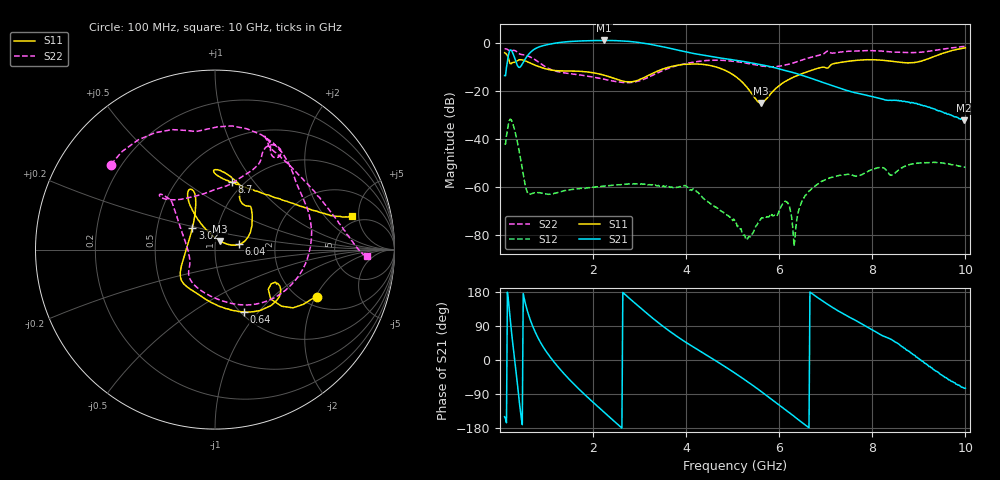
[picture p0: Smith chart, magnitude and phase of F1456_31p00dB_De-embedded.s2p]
! Integrated Device Technology
! Corporate Headquarters
! 6024 Silver Creek Valley Road
! San Jose, CA 95138  USA
! Phone:  1-408-284-8200
! Toll Free:  1-800-223-1366
! Webpage:  http://www.idt.com/
! Timing and RF Division
! 515 Groton Road, Suite 102
! Westford, MA 01886-6024
! Device:  F1456
! Description: 6-bit 0.5 dB Transmit Variable Gain Amplifier
! Frequency:  2100.0 -  2950.00 MHz
! Package:  6x6 mm Thin QFN Plastic Package: 28 pin
! State:  62
! Atten State:  31.0 dB
! Voltage:  +5.00 Volts
! Current:  216.927 mA
! Data:  The device was measured on a the F1455 evaluation board which has
!  individual transmission lines to the RF pins.  Data was collected
!  using a calibrated network analyzer.  The evaluation board was
!  de-embedded using a TRL calibration technique.
!  The reference plane is the edge of the package pin.
!  Pin  1 = CSb
!  Pin  2 = DATA
!  Pin  3 = CLK
!  Pin  4 = RSET
!  Pin  5 = GND
!  Pin  6 = RFIN  = Port 1
!  Pin  7 = GND
!  Pin  8 = NC
!  Pin  9 = NC
!  Pin 10 = NC
!  Pin 11 = NC
!  Pin 12 = NC
!  Pin 13 = NC
!  Pin 14 = /STBY
!  Pin 15 = GND
!  Pin 16 = RFOUT  = Port 2
!  Pin 17 = GND
!  Pin 18 = NC
!  Pin 19 = NC
!  Pin 20 = NC
!  Pin 21 = GND
!  Pin 22 = NC
!  Pin 23 = GND
!  Pin 24 = NC
!  Pin 25 = NC
!  Pin 26 = NC
!  Pin 27 = GND
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# GHz S dB R 50
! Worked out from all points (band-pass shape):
!   496 points, 100 MHz to 10 GHz, reference 50 ohm
!   highest |S21| = 1.01 dB at 2.24 GHz (marker M1); lowest = -32.3 dB at 9.96 GHz (marker M2)
!   |S21| within 3 dB of the highest: 802.1 MHz to 3.586 GHz (2.784 GHz wide, 127 % of centre)
!   lowest |S11| = -25.1 dB at 5.6 GHz (marker M3), VSWR 1.12, Z = 52.5 + j5.12 ohm
!   |S11| at or under -10 dB: 847.9 MHz to 3.656 GHz (2.809 GHz wide, 125 % of centre); 4.633 GHz to 7.071 GHz (2.439 GHz wide, 41.7 % of centre)
!   |S22| runs from -16.6 to -1.5 dB; largest |S21 - S12| = 1.1
!   S11 on the Smith chart (normalised r, x): 100 MHz: 2.37, -2.04; 640 MHz: 1.04, -0.84; 3.02 GHz: 0.75, +0.19; 6.04 GHz: 1.31, +0.08; 8.7 GHz: 0.89, +0.78; 10 GHz: 4.19, +4.17
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0.1  -4.10 -24.9  -13.67 -149.7  -42.29 50.5  -2.51 140.7
0.18  -6.25 -40.3  -5.42 159.6  -34.14 -2.4  -2.98 109.6
0.26  -8.34 -28.3  -3.62 60.4  -32.88 -100.9  -3.30 88.8
0.4  -7.17 -33.7  -10.15 -91.8  -43.83 148.7  -4.31 44.6
0.64  -8.33 -65.1  -4.24 109.9  -63.13 136.8  -5.79 -7.6
0.82  -9.82 -83.2  -1.84 57.9  -62.49 119.1  -7.88 -45.8
1.14  -11.47 -109.3  -0.27 -1.9  -63.02 88.7  -11.46 -91.4
1.76  -11.91 -137.5  0.82 -84.2  -60.70 57.1  -13.51 -132.6
2.24  -13.52 -153.1  1.01 -138.1  -59.79 41.8  -15.17 -145.3
3.02  -15.15 136.5  0.07 137.2  -58.98 12.2  -15.65 169.2
3.4  -11.68 114.5  -1.22 98.7  -59.49 -2.5  -12.45 145.4
4.1  -8.80 112.1  -4.22 38.7  -61.28 -37.1  -8.26 132.3
5.06  -13.99 119.7  -7.24 -35.5  -75.30 -73.1  -7.77 135.5
5.6  -25.09 60.7  -9.06 -81.9  -73.58 121.8  -9.57 121.4
6.04  -17.24 12.2  -11.07 -122.6  -68.24 113.4  -9.60 91.6
6.18  -15.55 15.2  -11.80 -135.5  -66.72 75.8  -9.00 81.7
6.32  -14.20 20.3  -12.50 -148.8  -84.87 95.5  -8.28 75.2
6.7  -11.42 39.5  -14.89 175.7  -60.82 133.2  -5.92 64.1
8.36  -7.53 89.5  -23.99 57.0  -54.66 48.1  -3.75 62.5
8.7  -8.26 75.8  -24.43 31.0  -51.48 58.5  -4.04 51.3
9.96  -2.19 13.6  -32.33 -73.3  -51.77 -30.1  -1.53 -2.3
10  -2.06 13.8  -32.19 -74.1  -51.84 -32.1  -1.46 -2.6
